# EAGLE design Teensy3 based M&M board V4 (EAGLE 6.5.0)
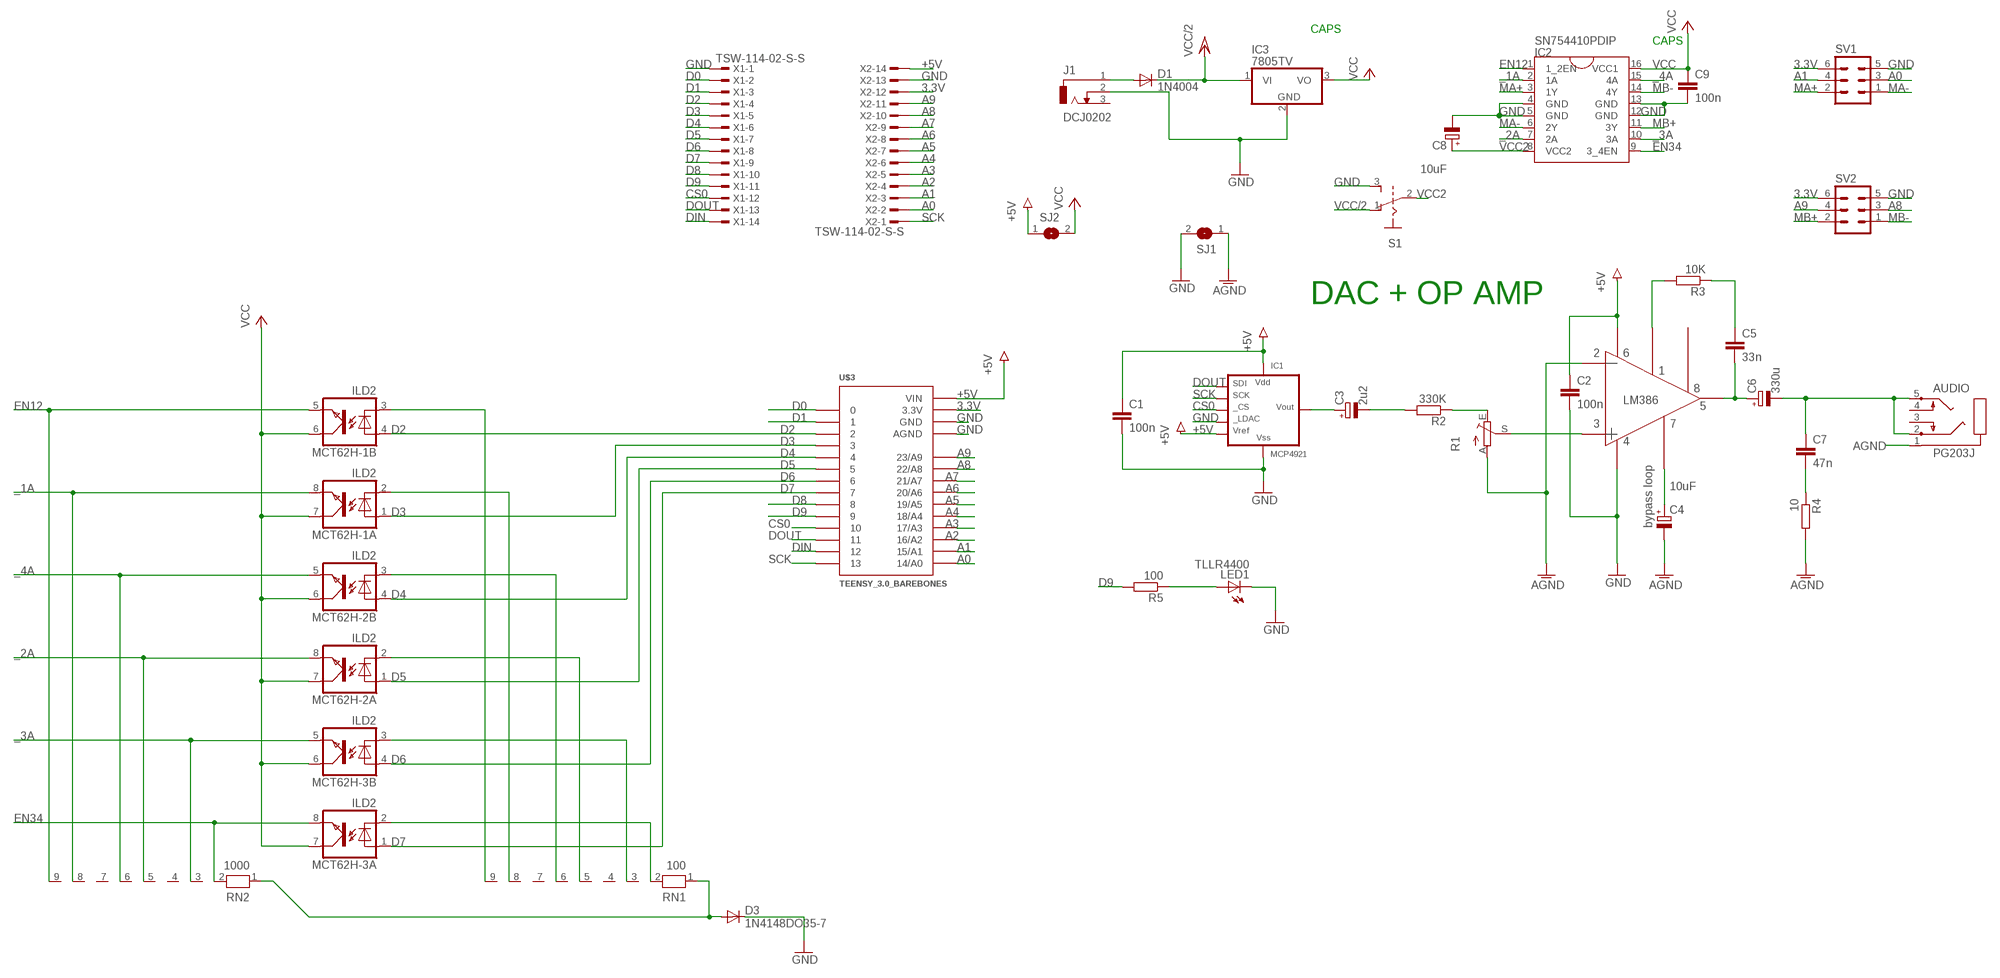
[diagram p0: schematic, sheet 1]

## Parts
AUDIO  PG203J  [PG203J]
C1  100n  C-EU050-030X075  [C050-030X075]
C2  100n  C-EU050-030X075  [C050-030X075]
C3  2u2  CPOL-EUE2-5  [E2-5]
C4  10uF  CPOL-EUE2-5  [E2-5]
C5  33n  C-EU050-030X075  [C050-030X075]
C6  330u  CPOL-EUE2.5-7  [E2,5-7]
C7  47n  C-EU050-030X075  [C050-030X075]
C8  10uF  CPOL-EUE2-5  [E2-5]
C9  100n  C-EU050-030X075  [C050-030X075]
D1  1N4004  [DO41-10]
D3  1N4148DO35-7  [DO35-7]
IC1  MCP4921  MCP4921P  [DIL8]
IC2  SN754410PDIP  [DIL16]
IC3  7805TV  [TO220V]
J1  DCJ0202  [DCJ0202]
LED1  TLLR4400  [LED3MM]
MCT62H-1  ILD2  [DIL08]
MCT62H-2  ILD2  [DIL08]
MCT62H-3  ILD2  [DIL08]
R1  TRIM_EU-CA9V  [CA9V]
R2  330K  R-EU_0207/10  [0207/10]
R3  10K  R-EU_0207/10  [0207/10]
R4  10  R-EU_0207/10  [0207/10]
R5  100  R-EU_0207/10  [0207/10]
RN1  100  RN08  [RN-9]
RN2  1000  RN08  [RN-9]
S1  EG1218  [GF-126-0159]
SJ1  SJ  [SJ]
SJ2  SJ  [SJ]
SV1  ML6  [ML6]
SV2  ML6  [ML6]
U$2  LM386  LM386OA  [LM386]
U$3  TEENSY_3.0_BAREBONES  [TEENSY_3.0_BAREBONES]
X1  TSW-114-02-S-S  [TSW-114-02-S-S]
X2  TSW-114-02-S-S  [TSW-114-02-S-S]

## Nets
3.3V [power]: SV1.6 SV2.6 U$3.3.3V X2.12
+5V [power]: C1.1 C2.1 IC1.1(VDD) IC1.6(VREF) SJ2.1 U$2.6 U$3.VIN X2.14
_1A: IC2.2(1A) MCT62H-1.8(A:EMIT) RN2.8
_2A: IC2.7(2A) MCT62H-2.8(A:EMIT) RN2.5
_3A: IC2.10(3A) MCT62H-3.5(B:EMIT) RN2.3
_4A: IC2.15(4A) MCT62H-2.5(B:EMIT) RN2.6
A0: SV1.3 U$3.14/A0 X2.2
A1: SV1.4 U$3.15/A1 X2.3
A2: U$3.16/A2 X2.4
A3: U$3.17/A3 X2.5
A4: U$3.18/A4 X2.6
A5: U$3.19/A5 X2.7
A6: U$3.20/A6 X2.8
A7: U$3.21/A7 X2.9
A8: SV2.3 U$3.22/A8 X2.10
A9: SV2.4 U$3.23/A9 X2.11
AGND [power]: AUDIO.1 C4.- R1.A R4.2 SJ1.1 U$2.2
AMP_IN: R1.S U$2.3
CS0: IC1.2(CS) U$3.10 X1.12
D0: U$3.0 X1.2
D1: U$3.1 X1.3
D2: MCT62H-1.4(B:A) U$3.2 X1.4
D3: MCT62H-1.1(A:A) U$3.3 X1.5
D4: MCT62H-2.4(B:A) U$3.4 X1.6
D5: MCT62H-2.1(A:A) U$3.5 X1.7
D6: MCT62H-3.4(B:A) U$3.6 X1.8
D7: MCT62H-3.1(A:A) U$3.7 X1.9
D8: U$3.8 X1.10
D9: R5.2 U$3.9 X1.11
DIN: U$3.12 X1.14
DOUT: IC1.4(SDI) U$3.11 X1.13
EN12: IC2.1(1_2EN) MCT62H-1.5(B:EMIT) RN2.9
EN34: IC2.9(3_4EN) MCT62H-3.8(A:EMIT) RN2.2
GND [power]: C1.2 C2.2 C8.- C9.2 D3.C IC1.5(LDAC) IC1.7(VSS) IC2.4(GND) IC2.5(GND) IC2.12(GND) IC2.13(GND) IC3.2(GND) J1.2 LED1.K(C) S1.3 SJ1.2 SV1.5 SV2.5 U$2.4 U$3.AGND U$3.GND X1.1 X2.13
MA+: IC2.3(1Y) SV1.2
MA-: IC2.6(2Y) SV1.1
MB+: IC2.11(3Y) SV2.2
MB-: IC2.14(4Y) SV2.1
N$1: D1.A J1.1
N$2: R3.2 U$2.1
N$3: C3.+ IC1.8(VOUT)
N$4: C3.- R2.2
N$5: LED1.A R5.1
N$6: R1.E R2.1
N$7: D3.A RN1.1 RN2.1
N$9: C5.1 R3.1
N$10: C4.+ U$2.7
N$13: MCT62H-3.2(A:C) RN1.2
N$14 [power]: MCT62H-1.3(B:C) RN1.9
N$16 [power]: MCT62H-1.2(A:C) RN1.8
N$17 [power]: MCT62H-2.3(B:C) RN1.6
N$18 [power]: MCT62H-2.2(A:C) RN1.5
N$19 [power]: MCT62H-3.3(B:C) RN1.3
N$78: C7.2 R4.1
N$84: AUDIO.2 AUDIO.5 C6.- C7.1
N$99: C5.2 C6.+ U$2.5
SCK: IC1.3(SCK) U$3.13 X2.1
VCC: C9.1 IC2.16(VCC1) IC3.3(VO) MCT62H-1.6(B:COL) MCT62H-1.7(A:COL) MCT62H-2.6(B:COL) MCT62H-2.7(A:COL) MCT62H-3.6(B:COL) MCT62H-3.7(A:COL) SJ2.2
VCC2: C8.+ IC2.8(VCC2) S1.2
VCC/2: D1.C IC3.1(VI) S1.1
Unconnected: AUDIO.3 AUDIO.4 J1.3 RN1.4 RN1.7 RN2.4 RN2.7 U$2.8

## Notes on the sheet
- CAPS
- CAPS
- DAC + OP AMP
- bypass loop

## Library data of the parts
AUDIO = con-hirschmann:PG203J: MIC/HEADPHONE JACK KS-S stereo microphone/headphone jack PG203JN (Schukat)
C1 C2 C5 C7 C9 = rcl:C-EU: CAPACITOR, European symbol
C3 C4 C6 C8 = rcl:CPOL-EU: POLARIZED CAPACITOR, European symbol
D1 = diode:1N4004: DIODE
D3 = diode:1N4148: DIODE
IC1 = microchip-dac:MCP4921: MCP4921: 12-bit DAC MCP4901/4911/4921 - 8/10/12-Bit Voltage Output Digital-to-Analog Converter with SPI Interface Interface The MCP49x1 devices are single channel 8-bit, 10-bit and 12-bit buffered voltage output Digital-to-Analog Converters (DACs), respectively. The devices operate from a single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
IC2 = AlexW-Eagle-Libraries:SN754410
IC3 = linear:78*: Positive VOLTAGE REGULATOR Source: http://cache.national.com/ds/LM/LM78L05.pdf http://www.fairchildsemi.com/ds/LM/LM7805.pdf
J1 = con-jack:DCJ0202: DC POWER JACK Source: DCJ0202.pdf; OC_FARNELL: unknown; OC_NEWARK: unknown
LED1 = led:TLLR4400: Low Current (2mA) LED 3 mm Tinted Diffused Package color RED; MF: VISHAY SEMICONDUCTOR; OC_FARNELL: 1612437
MCT62H-1-MCT62H-3 = optocoupler:ILD2: SIEMENS OPTO COUPLER; OC_FARNELL: 1469596; OC_NEWARK: unknown
R1 = pot:TRIM_EU-: POTENTIOMETER
R2-R5 = rcl:R-EU_: RESISTOR, European symbol
RN1 RN2 = resistor-net:RN08: RESISTOR NETWORK; OC_FARNELL: unknown; OC_NEWARK: unknown
S1 = videomusik:EG1218
SJ1 SJ2 = jumper:SJ: SMD solder JUMPER
SV1 SV2 = con-harting-ml:ML6: HARTING; OC_FARNELL: unknown; OC_NEWARK: unknown
U$2 = blushingboy_experimental:LM386
U$3 = Teensy3.0:TEENSY_3.0_BAREBONES
X1 X2 = con-samtec:TSW-114-02-S-S: THROUGH-HOLE .025" SQ POST HEADER Source: Samtec TSW.pdf; OC_FARNELL: unknown; OC_NEWARK: unknown

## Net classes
1 power: width 0.61 mm

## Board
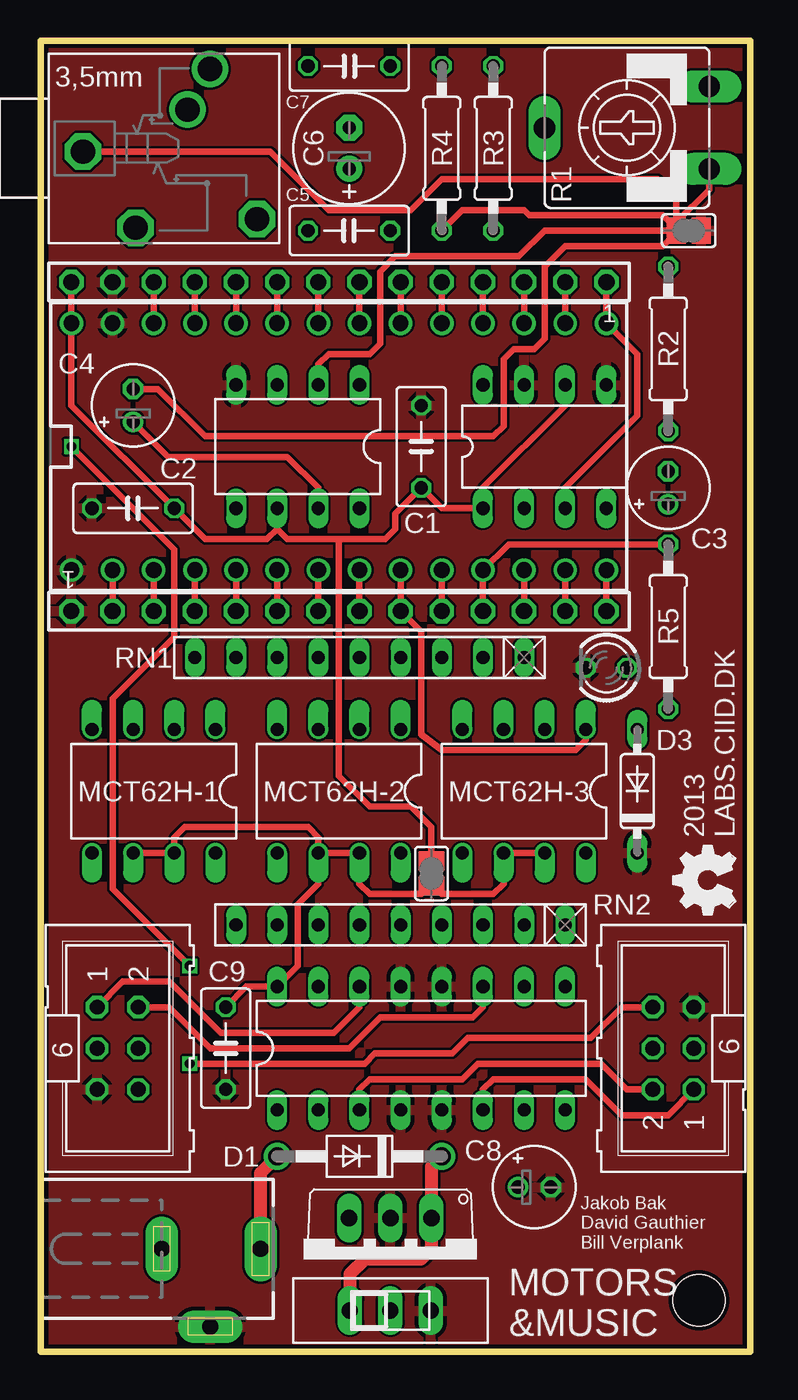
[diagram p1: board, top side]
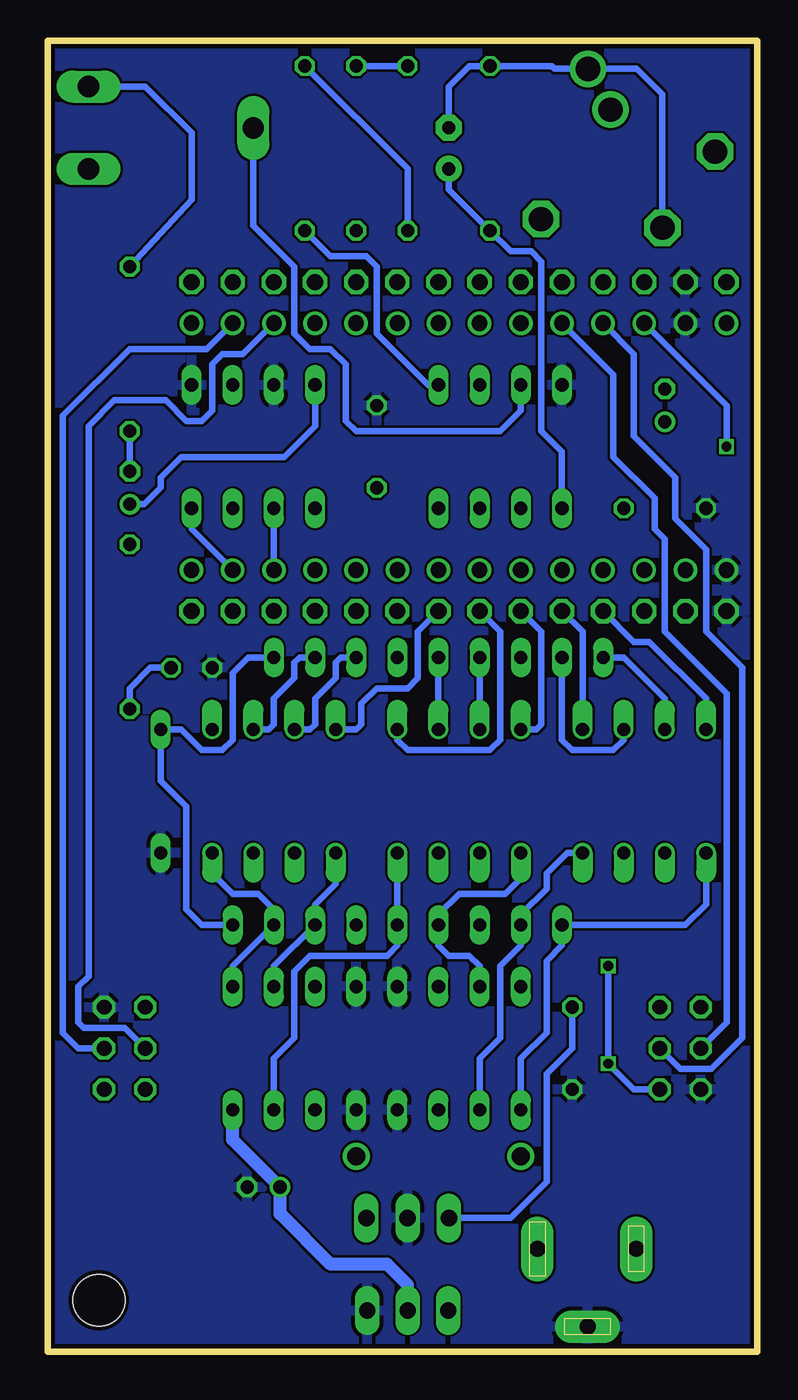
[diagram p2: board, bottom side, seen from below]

Size 43.8 x 80.95 mm. Coordinates in mm from the lower left corner, seen from the top.
Outline: 0,0 43.8,0 43.8,80.95 0,80.95 0,0
Copper layers (1*2*15*16): Top 0.035mm / dielectric 0.2mm / layer 2 0.0175mm / dielectric 1.1mm / layer 15 0.0175mm / dielectric 0.2mm / Bottom 0.035mm
Design rules "SeeedStudio_DRU_no_angle_20130527": minimum track width 6mil, minimum drill 12mil, track to track 6mil, track to pad 6mil, pad to pad 6mil, via to via 6mil, smd to smd 0mil, copper to edge 10mil, drill to drill 10mil, minimum pad ring 6mil, minimum via ring 6mil, stop-mask expansion 2mil, vias tented up to drill 25mil, thermal gap 10mil
Holes 3.2 mm at 40.64,3.17

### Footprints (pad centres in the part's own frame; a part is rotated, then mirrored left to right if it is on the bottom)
PG203J = drill 1.499 octagon: 1 -5.004,-0.203; 4 5.74,-4.369; 5 -1.753,-4.902 | drill 1.499: 2 2.845,4.902; 3 1.448,2.388
C050-030X075 = drill 0.813 octagon: 1 -2.54,0; 2 2.54,0
E2-5 = drill 0.813 pad 1.27: + -1.016,0 | drill 0.813 pad 1.27 octagon: - 1.016,0
E2,5-7 = drill 0.813 pad 1.6: + -1.27,0 | drill 0.813 pad 1.6 octagon: - 1.27,0
DO41-10 = drill 1.118: A 5.08,0; C -5.08,0
DO35-7 = drill 0.813 long: A 3.81,0; C -3.81,0
DIL8 = drill 0.813 long: 1 -3.81,-3.81; 2 -1.27,-3.81; 3 1.27,-3.81; 4 3.81,-3.81; 5 3.81,3.81; 6 1.27,3.81; 7 -1.27,3.81; 8 -3.81,3.81
DIL16 = drill 0.813 long: 1 -8.89,-3.81; 2 -6.35,-3.81; 3 -3.81,-3.81; 4 -1.27,-3.81; 5 1.27,-3.81; 6 3.81,-3.81; 7 6.35,-3.81; 8 8.89,-3.81; 9 8.89,3.81; 10 6.35,3.81; 11 3.81,3.81; 12 1.27,3.81; 13 -1.27,3.81; 14 -3.81,3.81; 15 -6.35,3.81; 16 -8.89,3.81
TO220V = drill 1.016 long: 1 -2.54,-2.54; 2 0,-2.54; 3 2.54,-2.54
DCJ0202 = drill 1 pad 2 long: 1 0,3.1; 2 4.8,0; 3 0,-3
LED3MM = drill 0.813 octagon: A -1.27,0; K 1.27,0
DIL08 = drill 0.813 offset: 1 -3.81,-3.81; 2 -1.27,-3.81; 3 1.27,-3.81; 4 3.81,-3.81; 5 3.81,3.81; 6 1.27,3.81; 7 -1.27,3.81; 8 -3.81,3.81
CA9V = drill 1.321 long: A -2.54,-5.08; E 2.54,-5.08; S 0,5.08
0207/10 = drill 0.813 octagon: 1 -5.08,0; 2 5.08,0
RN-9 = drill 0.813 long: 1 -10.16,0; 2 -7.62,0; 3 -5.08,0; 4 -2.54,0; 5 0,0; 6 2.54,0; 7 5.08,0; 8 7.62,0; 9 10.16,0
GF-126-0159 = drill 1 long: 1 -2.5,0; 2 0,0; 3 2.5,0
SJ = smd 1.168 x 1.6: 1 -0.762,0; 2 0.762,0
ML6 = drill 0.914 octagon: 1 -2.54,-1.27; 2 -2.54,1.27; 3 0,-1.27; 4 0,1.27; 5 2.54,-1.27; 6 2.54,1.27
LM386 = drill 0.813 long: 1 2.54,-2.54; 2 5.08,-2.54; 3 7.62,-2.54; 4 10.16,-2.54; 5 10.16,5.08; 6 7.62,5.08; 7 5.08,5.08; 8 2.54,5.08
TEENSY_3.0_BAREBONES = drill 0.965: 0 -7.62,13.97; 1 -7.62,11.43; 2 -7.62,8.89; 3 -7.62,6.35; 3.3V 7.62,11.43; 4 -7.62,3.81; 5 -7.62,1.27; 6 -7.62,-1.27; 7 -7.62,-3.81; 8 -7.62,-6.35; 9 -7.62,-8.89; 10 -7.62,-11.43; 11 -7.62,-13.97; 12 -7.62,-16.51; 13 7.62,-16.51; 14/A0 7.62,-13.97; 15/A1 7.62,-11.43; 16/A2 7.62,-8.89; 17/A3 7.62,-6.35; 18/A4 7.62,-3.81; 19/A5 7.62,-1.27; 20/A6 7.62,1.27; 21/A7 7.62,3.81; 22/A8 7.62,6.35; 23/A9 7.62,8.89; AGND 7.62,13.97; GND -7.62,16.51; VIN 7.62,16.51
TSW-114-02-S-S = drill 1 pad 1.5 octagon: 1 16.51,0; 2 13.97,0; 3 11.43,0; 4 8.89,0; 5 6.35,0; 6 3.81,0; 7 1.27,0; 8 -1.27,0; 9 -3.81,0; 10 -6.35,0; 11 -8.89,0; 12 -11.43,0; 13 -13.97,0; 14 -16.51,0

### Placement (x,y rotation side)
AUDIO  7.62,74.3 0 top
C1  23.5,55.88 90 top
C2  5.71,52.07 180 top
C3  38.73,53.34 90 top
C4  5.71,58.42 90 top
C5  19.05,69.22 180 top
C6  19.05,74.3 90 top
C7  19.05,79.38 0 top
C8  30.48,10.16 0 top
C9  11.43,18.73 270 top
D1  19.68,12.06 180 top
D3  36.83,34.61 90 top
IC1  31.11,55.88 0 top
IC2  23.5,18.73 0 top
IC3  21.59,5.71 180 top
J1  10.48,6.35 270 top
LED1  34.92,42.23 180 top
MCT62H-1  6.99,34.61 180 top
MCT62H-2  18.41,34.61 180 top
MCT62H-3  29.84,34.61 180 top
R1  36.2,75.56 90 top
R2  38.73,61.91 270 top
R3  27.94,74.3 270 top
R4  24.77,74.3 270 top
R5  38.73,44.77 90 top
RN1  19.68,42.86 180 top
RN2  22.23,26.35 180 top
S1  21.59,2.54 0 top
SJ1  40.01,69.22 0 top
SJ2  24.13,29.53 270 top
SV1  39.05,18.73 90 top
SV2  4.76,18.73 270 top
U$1  [OSHW_FILLX150_NOTEXT]  42.86,26.99 90 top
U$2  22.23,57.15 180 top
U$3  18.41,55.88 90 top
X1  18.41,45.72 180 top
X2  18.41,66.04 0 top

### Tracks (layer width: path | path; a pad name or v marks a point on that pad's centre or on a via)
3.3V  (via drill 0.6)
  Top 0.406: X2.12 U$3.3.3V | v1.91,55.88 8.26,49.53 8.26,44.13 4.45,40.32 4.45,28.57 v9.21,23.81 | SV1.6 35.88,21.27 33.97,19.37 26.35,19.37 25.4,18.41 20.64,18.41 20,17.78 v9.21,17.78
  Bottom 0.406: U$3.3.3V 1.91,58.42 v1.91,55.88 | SV2.6 7.62,16.19 v9.21,17.78 v9.21,23.81
+5V
  Top 0.406: X2.14 U$3.VIN 1.91,58.42 C2.1 10.16,50.16 13.97,50.16 14.61,50.8 | IC1.6 32.38,58.42 27.3,53.34 IC1.1 24.77,52.07 C1.1 21.91,51.75 21.91,50.8 21.27,50.16 18.41,50.16 | 14.61,50.8 U$2.6 | 18.41,50.16 15.24,50.16 14.61,50.8 | 18.41,50.16 18.41,35.56 20.32,33.66 22.86,33.66 24.13,32.38 SJ2.1 24.13,28.57
_1A
  Bottom 0.406: MCT62H-1.8 11.75,30.8 13.02,29.53 13.02,28.57 14.61,26.99 RN2.8 14.61,25.08 15.88,23.81 15.88,19.37 17.14,18.1 IC2.2
_2A
  Bottom 0.406: MCT62H-2.8 RN2.5 22.23,25.08 22.86,24.45 27.62,24.45 28.57,23.5 28.57,19.37 29.84,18.1 IC2.7
_3A
  Bottom 0.406: MCT62H-3.5 26.04,28.89 27.3,27.62 RN2.3 29.84,23.81 IC2.10
_4A
  Bottom 0.406: MCT62H-2.5 14.61,29.21 15.56,28.26 18.41,28.26 19.68,26.99 RN2.6 19.68,25.08 19.05,24.45 17.78,24.45 17.14,23.81 IC2.15
A0
  Top 0.406: X2.2 U$3.14/A0
  Bottom 0.406: U$3.14/A0 33.97,61.91 38.73,61.91 42.86,57.78 42.86,19.68 41.91,18.73 SV1.3
A1
  Top 0.406: X2.3 U$3.15/A1
  Bottom 0.406: U$3.15/A1 31.75,61.59 33.02,61.59 33.66,60.96 33.66,58.1 34.29,57.47 35.24,57.47 36.51,58.74 39.69,58.74 41.27,57.15 41.27,23.18 41.91,22.54 41.91,20.32 41.59,20 39.05,20 SV1.4
A2
  Top 0.406: X2.4 U$3.16/A2
A3
  Top 0.406: X2.5 U$3.17/A3
A4
  Top 0.406: X2.6 U$3.18/A4
A5
  Top 0.406: X2.7 U$3.19/A5
A6
  Top 0.406: X2.8 U$3.20/A6
A7
  Top 0.406: X2.9 U$3.21/A7
A8
  Top 0.406: X2.10 U$3.22/A8
  Bottom 0.406: U$3.22/A8 8.89,60.33 8.89,55.24 6.35,52.7 6.35,50.8 5.71,50.16 5.71,44.45 1.91,40.64 1.91,20.32 SV2.3
A9
  Top 0.406: X2.11 U$3.23/A9
  Bottom 0.406: U$3.23/A9 7.62,61.59 7.62,56.52 5.08,53.98 5.08,51.44 3.17,49.53 3.17,44.45 0.95,42.23 0.95,19.37 2.86,17.46 4.76,17.46 SV2.4
AGND
  Top 0.406: AUDIO.1 14.17,74.09 17.78,70.48 22.86,70.48 24.77,72.39 38.1,72.39 39.24,71.25 SJ1.1 | U$2.2 17.14,60.96 17.78,61.59 20.32,61.59 20.95,62.23 20.95,66.67 21.91,67.63 29.53,67.63 31.11,69.22 SJ1.1 | C4.- 7.24,59.44 10.16,56.52 27.94,56.52 28.57,57.15 28.57,61.28 29.21,61.91 30.48,61.91 31.11,62.55 31.11,66.99 32.38,68.26 38.42,68.26 39.24,69.09 SJ1.1 | 40.64,69.22 SJ1.1 | R4.2 26.04,70.48 29.84,70.48 30.16,70.17 38.42,70.17 39.24,69.34 SJ1.1 | R1.A 41.27,71.75 39.24,69.72 SJ1.1
AMP_IN
  Bottom 0.406: U$2.3 14.61,58.1 15.88,56.83 24.77,56.83 25.4,57.47 25.4,60.96 26.35,61.91 27.62,61.91 28.57,62.87 28.57,66.99 31.11,69.53 R1.S
CS0
  Top 0.406: U$3.10 X1.12
  Bottom 0.406: U$3.10 IC1.2
D0
  Top 0.406: U$3.0 X1.2
D1
  Top 0.406: U$3.1 X1.3
D2
  Top 0.406: U$3.2 X1.4
  Bottom 0.406: MCT62H-1.4 3.17,40.32 6.67,43.81 7.62,43.81 X1.4
D3
  Top 0.406: U$3.3 X1.5
  Bottom 0.406: MCT62H-1.1 10.79,44.45 X1.5
D4
  Top 0.406: U$3.4 X1.6
  Bottom 0.406: MCT62H-2.4 13.65,38.42 13.34,38.73 13.34,44.45 X1.6
D5
  Top 0.406: U$3.5 X1.7
  Bottom 0.406: MCT62H-2.1 22.23,37.78 21.59,37.15 16.51,37.15 15.88,37.78 15.88,44.45 X1.7
D6
  Top 0.406: U$3.6 X1.8
  Bottom 0.406: MCT62H-3.4 24.77,38.42 24.45,38.73 24.45,40.01 23.5,40.96 21.59,40.96 20.95,41.59 20.95,44.45 X1.8
D7
  Top 0.406: MCT62H-3.1 33.66,37.78 33.02,37.15 24.77,37.15 23.5,38.1 23.5,44.45 X1.9 U$3.7
D8
  Top 0.406: U$3.8 X1.10
D9
  Top 0.406: X1.11 U$3.9 28.89,49.85 R5.2
DIN
  Top 0.406: U$3.12 X1.14
DOUT
  Top 0.406: U$3.11 X1.13
  Bottom 0.406: U$3.11 34.92,50.8 IC1.4
EN12
  Bottom 0.406: MCT62H-1.5 3.17,27.62 4.45,26.35 RN2.9 12.06,25.08 13.02,24.13 13.02,19.68 14.61,18.1 IC2.1
EN34
  Bottom 0.406: MCT62H-3.8 33.66,29.53 32.38,28.26 30.8,28.26 29.84,27.3 RN2.2 32.38,23.81 IC2.9
GND
  pour Bottom: -1.91,-0.95 -1.91,82.23 50.8,82.23 50.8,-0.95
  pour Top: -0.95,81.6 -0.95,-0.95 50.8,-0.95 50.8,81.6
MA+
  Top 0.406: IC2.3 19.68,16.19 20.32,16.83 26.04,16.83 26.99,17.78 34.61,17.78 36.2,16.19 SV1.2
MA-
  Top 0.406: IC2.6 27.3,16.19 27.94,16.83 33.66,16.83 35.88,14.61 38.73,14.61 SV1.1
MB+
  Top 0.406: IC2.11 27.3,21.27 26.67,20.64 20.95,20.64 19.05,18.73 10.48,18.73 7.94,21.27 SV2.2
MB-
  Top 0.406: IC2.14 19.68,21.27 18.1,19.68 11.11,19.68 7.94,22.86 5.08,22.86 SV2.1
N$1
  Top 0.813: J1.1 13.58,11.04 D1.A
N$2
  Bottom 0.406: U$2.1 20.32,59.69 23.5,62.87 23.5,66.99 24.13,67.63 26.35,67.63 R3.2
N$3
  Bottom 0.406: IC1.8 27.3,57.15 29.21,55.24 35.56,55.24 36.83,53.98 36.83,53.34 37.85,52.32 C3.+
N$4
  Bottom 0.406: R2.2 C3.-
N$5
  Bottom 0.406: R5.1 38.73,40.96 37.47,42.23 LED1.A
N$6
  Bottom 0.406: R2.1 34.92,71.12 34.92,75.25 37.78,78.11 R1.E
N$7
  Bottom 0.406: RN1.1 31.43,42.86 32.38,41.91 32.38,37.78 33.02,37.15 34.29,37.15 35.56,38.42 D3.A 36.83,35.24 35.24,33.66 35.24,27.3 34.29,26.35 RN2.1
N$9
  Bottom 0.406: C5.1 21.59,73.03 R3.1
N$10
  Top 0.406: U$2.7 17.14,53.34 15.24,55.24 7.87,55.24 C4.+
N$13
  Bottom 0.406: MCT62H-3.2 30.16,38.42 29.84,38.73 29.84,40.32 28.57,41.59 28.57,42.55 28.26,42.86 RN1.2
N$14
  Bottom 0.406: RN1.9 8.26,42.86 5.71,40.32 MCT62H-1.3
N$16
  Bottom 0.406: MCT62H-1.2 8.26,37.78 8.89,37.15 11.43,37.15 12.06,37.78 RN1.8
N$17
  Bottom 0.406: MCT62H-2.3 RN1.6
N$18
  Bottom 0.406: RN1.5 MCT62H-2.2
N$19
  Bottom 0.406: MCT62H-3.3 27.62,38.42 27.3,38.73 27.3,40.32 26.04,41.59 26.04,42.55 25.72,42.86 RN1.3
N$78
  Bottom 0.406: C7.2 R4.1
N$84
  Bottom 0.406: C6.- 19.05,78.11 17.78,79.38 C7.1 12.7,79.38 12.52,79.2 AUDIO.2 7.44,79.2 5.87,77.62 AUDIO.5
N$99
  Bottom 0.406: C6.+ 19.05,71.75 C5.2 15.24,67.94 13.97,67.94 13.34,67.31 13.34,56.83 12.06,55.56 U$2.5
SCK
  Top 0.406: X2.1 U$3.13 36.83,61.59 36.83,57.78 32.38,53.34 IC1.3
VCC
  Top 0.406: MCT62H-3.7 MCT62H-3.6 28.57,28.89 27.94,28.26 24.77,28.26 24.26,28.77 SJ2.2 24,28.77 23.5,28.26 20.32,28.26 19.68,28.89 MCT62H-2.7 MCT62H-2.6 | MCT62H-2.6 17.14,31.75 16.51,32.38 8.89,32.38 8.26,31.75 MCT62H-1.7 MCT62H-1.6 | MCT62H-2.6 17.14,28.89 15.88,27.62 15.88,23.81 IC2.16 12.7,22.54 C9.1
  Bottom 0.406: IC3.3 15.24,8.26 13.02,10.48 13.02,17.14 11.43,18.73 C9.1
VCC2
  Bottom 0.813: S1.2 21.59,4.13 22.86,5.4 26.35,5.4 29.46,8.51 C8.+ 32.38,13.08 IC2.8
VCC/2
  Top 0.813: D1.C 24.13,11.43 IC3.1 24.13,6.35 23.5,5.71 20,5.71 19.09,4.8 S1.1

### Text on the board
tNames: 2013 / LABS.CIID.DK | Jakob Bak / David Gauthier / Bill Verplank | MOTORS / &MUSIC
